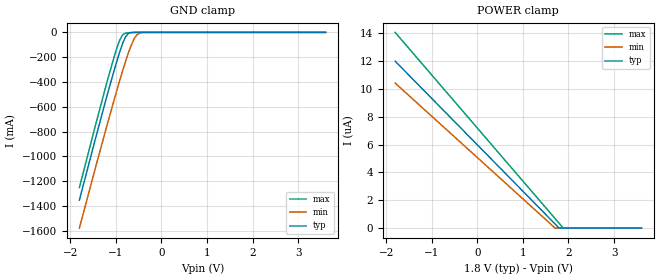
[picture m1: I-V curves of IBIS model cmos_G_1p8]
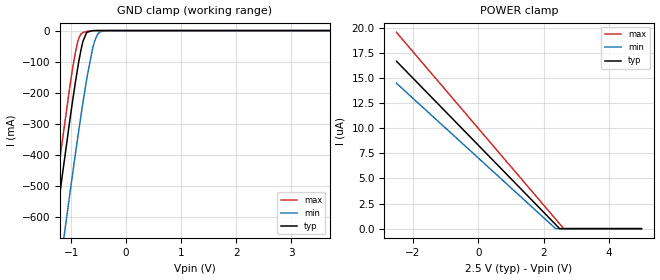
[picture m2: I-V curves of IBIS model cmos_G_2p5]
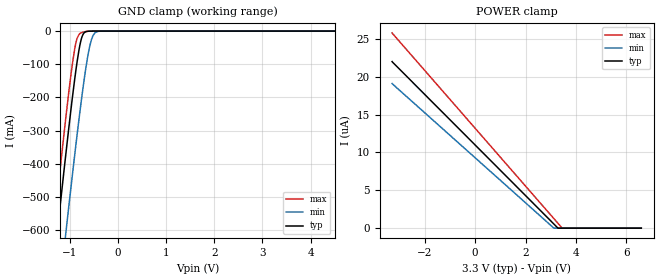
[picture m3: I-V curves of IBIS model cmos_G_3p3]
|Texas Instruments Incorporated
| 1.8V, 2.5V, 3.3V LVCMOS High-Performance Clock Buffer
| Marketing Part # : LMK1C1108
| Voltage Range : 1.71V-3.465V
| Package-type: TSSOP
| #pins/pkg drawing : 16-pin TSSOP
[IBIS Ver] 1.0
[File name] lmk1c1108.ibs
[File Rev] 1.0
[Date] 11/25/2020
[Source]
| Texas Instruments Incorporated.
| 12500 TI Blvd
| Dallas, TX -75243
[Notes] Revision History:
| Rev 1.0: 11/25/2020
| - Initial version of the model
| - Model generated from simulations in SPECTRE
| - C_comp although listed in numerical order of value are
| obtained from varying PVT conditions. For PVT conditions for
| each specific value refer the buffer description under
| respective [Model]. IBIS model user is responsible for using
| appropriate C_comp to simulate for Signal Integrity.
| - Warnings regarding combined Non-monotonicity of various models have been
| reviewed and considered minor and can be ignored.
| - Model names with a trailing _1p8 contain the model for
| 1.8V operation. Model names with a trailing _2p5 contain the model
| for 2.5V operation. Model names with a trailing _3p3 contain the model
| for 3.3V operation.
[Disclaimer]
| This model is designed as an aid for customers of Texas Instruments.
| TI and its licensors and suppliers make no warranties, either expressed
| or implied, with respect to this model, including the warranties of
| merchantability or fitness for a particular purpose. The model is
| provided solely on an "as is" basis. The entire risk as to its quality
| and performance is with the customer.
| This model is subject to change without notice. Texas Instruments
| Incorporated is not responsible for updating this model.
[Copyright]
(C) Copyright 2020 Texas Instruments Incorporated. All rights reserved.
|   Component LMK1C1108
[Component]   LMK1C1108
[Manufacturer]  Texas Instruments Incorporated
[Package] |16-pin TSSOP package
| variable   typ   min   max
R_pkg   35m   28m   80m
L_pkg   3.2n   2.6n   3.8n
C_pkg   0.35p   0.28p   0.41p
|-------------------------PIN------------------------------------------------
[Pin]  signal_name   model_name   R_pin   L_pin   C_pin
1   CLKIN   cmos_in   32.54m   3.6n   0.35p
2   1G   cmos_G   80.4m   3.27n   0.335p
3   Y0   cmos_out   39.39m   3.05n   0.324p
4   GND   GND   36.48m   2.897n   0.328p
5   VDD   POWER   24.25m   2.5n   0.353p
6   Y4   cmos_out   38.37m   3.02n   0.326p
7   GND   GND   39.73m   3.245n   0.38p
8   Y6   cmos_out   31.16m   3.72n   0.34p
9   Y7   cmos_out   32.6m   3.585n   0.355p
10   VDD   POWER   41.12m   3.31n   0.389p
11   Y5   cmos_out   40.33m   3.10n   0.334p
12   GND   GND   36.77m   2.93n   0.329p
13   Y2   cmos_out   36.28m   2.884n   0.326p
14   VDD   POWER   38.56m   3.012n   0.324p
15   Y3   cmos_out   39.74m   3.257n   0.38p
16   Y1   cmos_out   34.18m   3.725n   0.362p
[Model Selector]   cmos_in
cmos_in_1p8   cmos input model at 1.8V
cmos_in_2p5   cmos input model at 2.5V
cmos_in_3p3   cmos input model at 3.3V
[Model Selector]   cmos_G
cmos_G_1p8   cmos 1G model at 1.8V
cmos_G_2p5   cmos 1G model at 2.5V
cmos_G_3p3   cmos 1G model at 3.3V
[Model Selector]   cmos_out
cmos_out_1p8   cmos output model at 1.8V
cmos_out_2p5   cmos output model at 2.5V
cmos_out_3p3   cmos output model at 3.3V
| Models and submodels in the file (9): cmos_G_1p8 (Input), cmos_G_2p5 (Input), cmos_G_3p3 (Input), cmos_in_1p8 (Input), cmos_in_2p5 (Input), cmos_in_3p3 (Input), cmos_out_1p8 (Output), cmos_out_2p5 (Output), cmos_out_3p3 (Output)
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[Model]   cmos_G_1p8
Model_type   Input
Vinl = 0.45
Vinh = 1.35
|   typ   min   max
C_comp   2.69pF   2.601pF   2.886pF
[Voltage Range]   1.8   1.71   1.89
[Temperature Range]   25   150   -40
[Power Clamp Reference]   1.8   1.71   1.89
[GND Clamp Reference]   0   0   0
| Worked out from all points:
|   GND clamp passes 1 mA (typ) near -0.62 V on its own axis
[GND Clamp]
|   Voltage   I(typ)   I(min)   I(max)
-1.8V     -1.351A    -1.577A    -1.251A
-1.211V   -533.8mA   -771.9mA   -423.2mA
-1.039V   -307.6mA   -544.8mA   -198.6mA
-925.2mV  -169.5mA   -400.5mA   -72.4mA
-844.2mV  -83.24mA   -301.1mA   -17.85mA
-784.8mV  -34.97mA   -231.3mA   -6.505mA
-725.4mV  -8.825mA   -165.5mA   -3.073mA
-601.2mV  -280.2uA   -52.64mA   -316uA
-531mV    -45.76uA   -16.45mA   -52.62uA
-444.6mV  -5.415uA   -2.134mA   -5.055uA
-342mV    -1.279uA   -137.3uA   -1.351uA
3.6V      0A         0A         0A
[POWER Clamp]
|   Voltage   I(typ)   I(min)   I(max)
-1.8V     12uA       10.43uA    14.07uA
1.699V    319.7nA    16.08nA    712.2nA
1.791V    13.1nA     0A         361.8nA
1.883V    0A         0A         11.28nA
3.6V      0A         0A         0A
[Model]   cmos_G_2p5
Model_type   Input
Vinl = 0.625
Vinh = 1.875
|   typ   min   max
C_comp   2.623pF   2.472pF   2.811pF
[Voltage Range]   2.5   2.375   2.625
[Temperature Range]   25   150   -40
[Power Clamp Reference]   2.5   2.375   2.625
[GND Clamp Reference]   0   0   0
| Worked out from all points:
|   GND clamp passes 1 mA (typ) near -0.63 V on its own axis
[GND Clamp]
|   Voltage   I(typ)   I(min)   I(max)
-2.5V     -2.35A     -2.56A     -2.262A
-1.48V    -901.5mA   -1.135A    -794.9mA
-1.232V   -562.1mA   -800.1mA   -451.7mA
-1.157V   -462mA     -700.4mA   -351.1mA
-1.022V   -287.3mA   -524mA     -179.1mA
-925mV    -169.3mA   -400.2mA   -72.21mA
-857.5mV  -96.2mA    -317.1mA   -23.38mA
-782.5mV  -33.5mA    -228.7mA   -6.31mA
-707.5mV  -5.337mA   -146.7mA   -2.398mA
-587.5mV  -196.1uA   -43.59mA   -227.3uA
-430mV    -3.965uA   -1.456mA   -3.623uA
5V        0A         0A         0A
[POWER Clamp]
|   Voltage   I(typ)   I(min)   I(max)
-2.5V     16.67uA    14.48uA    19.54uA
2.36V     444.4nA    22.36nA    989.6nA
2.487V    18.24nA    0A         502.7nA
2.615V    0A         0A         15.69nA
5V        0A         0A         0A
[Model]   cmos_G_3p3
Model_type   Input
Vinl = 0.825
Vinh = 2.475
|   typ   min   max
C_comp   2.566pF   2.41pF   2.75pF
[Voltage Range]   3.3   3.135   3.465
[Temperature Range]   25   150   -40
[Power Clamp Reference]   3.3   3.135   3.465
[GND Clamp Reference]   0   0   0
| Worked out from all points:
|   GND clamp passes 1 mA (typ) near -0.65 V on its own axis
[GND Clamp]
|   Voltage   I(typ)   I(min)   I(max)
-3.3V     -3.502A    -3.695A    -3.427A
-1.429V   -830.6mA   -1.065A    -723.1mA
-1.3V     -653.8mA   -891mA     -544.2mA
-1.28V    -626.9mA   -864.3mA   -517mA
-1.211V   -533.4mA   -771.5mA   -422.8mA
-1.102V   -389.4mA   -627.6mA   -278.9mA
-1.033V   -300.4mA   -537.4mA   -191.7mA
-904.2mV  -145.7mA   -374.3mA   -53.93mA
-765.6mV  -23.82mA   -209.5mA   -5.096mA
-587.4mV  -195.6uA   -43.53mA   -226.7uA
-419.1mV  -3.199uA   -1.092mA   -2.912uA
6.6V      0A         0A         0A
[POWER Clamp]
|   Voltage   I(typ)   I(min)   I(max)
-3.3V     22uA       19.11uA    25.8uA
3.115V    587nA      29.49nA    1.307uA
3.284V    24.16nA    0A         663.9nA
3.452V    0A         0A         20.76nA
6.6V      0A         0A         0A
